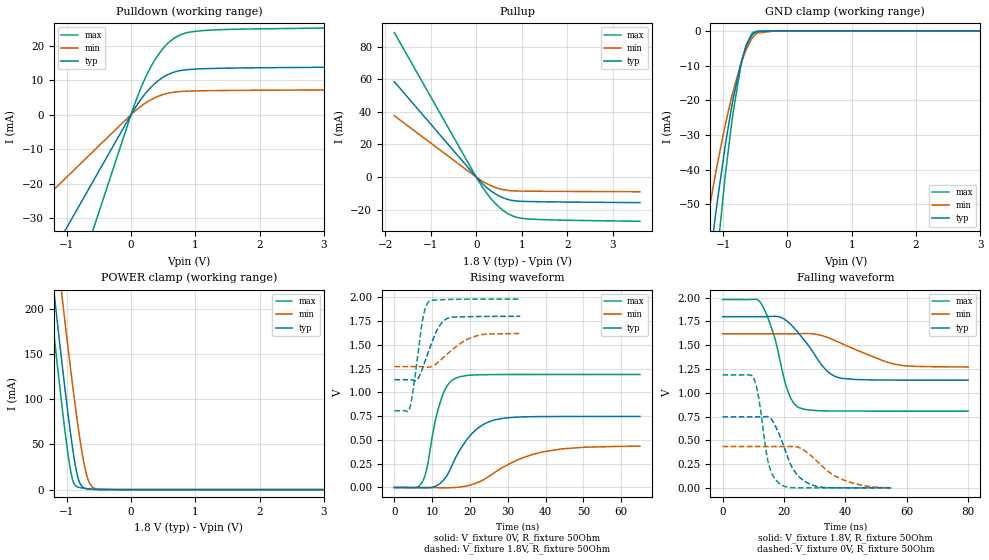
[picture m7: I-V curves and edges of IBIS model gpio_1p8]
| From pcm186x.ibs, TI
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|   gpio_1p8 Model
[Model]   gpio_1p8
Model_type   I/O
Polarity   Non-Inverting
Enable   Active-High
Vinl = 0.54
Vinh = 1.26
Vmeas = 0.9
Vref = 0
Cref = 2pF
Rref = 150
|   typ   min   max
|   (nom PVT)   (fast PVT)   (slow PVT)
C_comp   7.621e-12   7.539e-12   7.746e-12
[Model spec]
|subparameter
Vinl   0.54   0.486   0.594
Vinh   1.26   1.134   1.386
| Where nom  PVT is Nominal Process, 1.8V, 27C
|   Fast PVT is Strong Process,  1.98V, -40C
|   Slow PVT is Weak Process,   1.62V, 125C
[Voltage Range]   1.8   1.62   1.98
|Junction Temperature
[Temperature Range]   27   125   -40
[Pullup Reference]   1.8   1.62   1.98
[Pulldown Reference]   0   0   0
[Power Clamp Reference]   1.8   1.62   1.98
[GND Clamp Reference]   0   0   0
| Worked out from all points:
|   slope of the pulldown table from 0 to 0.27 V, typ, clamps not added: 37.8 ohm
|   slope of the pullup table from 0 to 0.27 V, typ, clamps not added: 37 ohm
|   GND clamp passes 1 mA (typ) near -0.54 V on its own axis
|   POWER clamp passes 1 mA (typ) near -0.68 V on its own axis
|   falling waveform, V_fixture 1.8V, R_fixture 50Ohm: 20-80 % time 9.26ns typ, 15.4ns min, 5.75ns max; typ from 1.8 V to 1.13 V
|   rising waveform, V_fixture 0V, R_fixture 50Ohm: 20-80 % time 7.07ns typ, 12.8ns min, 3.78ns max; typ from 0 V to 0.747 V
|   rising waveform, V_fixture 1.8V, R_fixture 50Ohm: 20-80 % time 3.89ns typ, 6.67ns min, 2.37ns max; typ from 1.13 V to 1.8 V
|   falling waveform, V_fixture 0V, R_fixture 50Ohm: 20-80 % time 6.04ns typ, 10.6ns min, 3.35ns max; typ from 0.747 V to 0 V
[Pulldown]
|   Voltage   I(typ)   I(min)   I(max)
-1.8V     -59mA      -32.59mA   -101.9mA
-33.84mV  -1.109mA   -612.7uA   -1.916mA
132.5mV   3.905mA    2.142mA    6.795mA
216.9mV   5.997mA    3.28mA     10.46mA
308.7mV   7.932mA    4.321mA    13.88mA
403.7mV   9.576mA    5.188mA    16.83mA
500.8mV   10.89mA    5.857mA    19.27mA
599.8mV   11.86mA    6.325mA    21.17mA
688.3mV   12.45mA    6.581mA    22.4mA
898.9mV   13.09mA    6.835mA    23.9mA
1.307V    13.43mA    6.987mA    24.59mA
3.6V      13.84mA    7.225mA    25.25mA
[GND Clamp]
|   Voltage   I(typ)   I(min)   I(max)
-1.8V     -261.5mA   -162.9mA   -369.6mA
-1.25V    -73.27mA   -54.97mA   -97.87mA
-1.128V   -54.43mA   -42.09mA   -71.54mA
-1.107V   -51.44mA   -40.02mA   -67.37mA
-972.4mV  -33.61mA   -27.55mA   -42.63mA
-871.7mV  -22.31mA   -19.4mA    -27.17mA
-726.8mV  -9.566mA   -9.704mA   -10.32mA
-642.6mV  -4.455mA   -5.402mA   -4.054mA
-529.2mV  -809.7uA   -1.62mA    -429.6uA
-473.2mV  -233.7uA   -687.4uA   -86.17uA
-180mV    -64.28nA   -820.8nA   -79.79nA
3.6V      0A         0A         0A
[Pullup]
|   Voltage   I(typ)   I(min)   I(max)
-1.8V     58.47mA    37.57mA    88.63mA
54mV      -1.661mA   -1.057mA   -2.54mA
156.2mV   -4.532mA   -2.867mA   -6.98mA
304.4mV   -8.057mA   -5.04mA    -12.56mA
469.1mV   -11.09mA   -6.833mA   -17.56mA
581.9mV   -12.64mA   -7.683mA   -20.27mA
724mV     -13.96mA   -8.326mA   -22.85mA
853.2mV   -14.61mA   -8.559mA   -24.4mA
1.115V    -14.98mA   -8.674mA   -25.66mA
1.98V     -15.36mA   -8.836mA   -26.53mA
3.6V      -15.71mA   -9.02mA    -27.16mA
[POWER Clamp]
|   Voltage   I(typ)   I(min)   I(max)
-1.8V     623.7mA    688.3mA    587.1mA
-1.403V   354.1mA    425.1mA    310.3mA
-1.189V   213.4mA    287.1mA    166.4mA
-1.099V   156mA      230.4mA    108.5mA
-1.051V   126.5mA    200.8mA    79.19mA
-931.7mV  57.79mA    129.3mA    18.15mA
-829.8mV  14.42mA    73.33mA    2.879mA
-761.6mV  3.259mA    41.06mA    1.751mA
-683.3mV  1.014mA    14.39mA    940.6uA
-607.7mV  454.4uA    3.109mA    396.4uA
-508.9mV  103.9uA    361.3uA    60.2uA
3.6V      0A         0A         0A
[Ramp]
R_load = 50
|   typ   min   max
dV/dt_r   0.448065/7.05531e-09   0.260737/1.27942e-08   0.712735/3.77208e-09
dV/dt_f   0.400024/9.2477e-09   0.209339/1.53703e-08   0.703487/5.72437e-09
[Falling Waveform]
V_fixture = 1.8V
V_fixture_min = 1.62V
V_fixture_max = 1.98V
R_fixture = 50Ohm
|   Time   V(typ)   V(min)   V(max)
0s        1.8V       1.62V      1.98V
12.43ns   1.8V       1.62V      1.945V
16.97ns   1.804V     1.62V      1.58V
21.37ns   1.743V     1.62V      1.007V
23.08ns   1.688V     1.62V      894.8mV
25.02ns   1.616V     1.621V     841.9mV
32.67ns   1.276V     1.598V     810mV
37.15ns   1.165V     1.542V     808.1mV
55.79ns   1.134V     1.301V     807.5mV
79.98ns   1.133V     1.271V     807.5mV
[Rising Waveform]
V_fixture = 0V
V_fixture_min = 0V
V_fixture_max = 0V
R_fixture = 50Ohm
|   Time   V(typ)   V(min)   V(max)
0s        930.6pV    43nV       571.3pV
7.3ns     -3.183mV   62.76uV    50.86mV
8.73ns    -3.524mV   289.9uV    221.7mV
10.58ns   8.717mV    -1.38mV    655.1mV
12.57ns   58.69mV    -2.413mV   949.2mV
16.26ns   317.5mV    350.4uV    1.15V
21.29ns   596.3mV    41.09mV    1.183V
27.85ns   722mV      191.9mV    1.187V
39.06ns   745.5mV    372.8mV    1.188V
64.95ns   746.8mV    434.6mV    1.188V
[Rising Waveform]
V_fixture = 1.8V
V_fixture_min = 1.62V
V_fixture_max = 1.98V
R_fixture = 50Ohm
|   Time   V(typ)   V(min)   V(max)
0s        1.133V     1.271V     807.5mV
4.04ns    1.134V     1.271V     830.5mV
4.74ns    1.132V     1.271V     966.6mV
6.07ns    1.134V     1.271V     1.349V
7.59ns    1.268V     1.271V     1.786V
9.25ns    1.453V     1.265V     1.958V
11.4ns    1.662V     1.31V      1.972V
13.9ns    1.776V     1.4V       1.976V
21.28ns   1.797V     1.589V     1.98V
33.3ns    1.8V       1.619V     1.98V
[Falling Waveform]
V_fixture = 0V
V_fixture_min = 0V
V_fixture_max = 0V
R_fixture = 50Ohm
|   Time   V(typ)   V(min)   V(max)
0s        746.8mV    434.6mV    1.188V
10.05ns   746.8mV    434.6mV    1.158V
11.7ns    746.8mV    434.6mV    960.1mV
14.1ns    748.9mV    434.6mV    404.4mV
15.15ns   744.9mV    434.6mV    231.8mV
19.29ns   494.3mV    434.6mV    29.31mV
23.65ns   164mV      433.1mV    1.317mV
28.63ns   37.33mV    342.8mV    219.9uV
39.01ns   533.1uV    87.92mV    74.38uV
54.9ns    61.48uV    1.022mV    54.09uV
